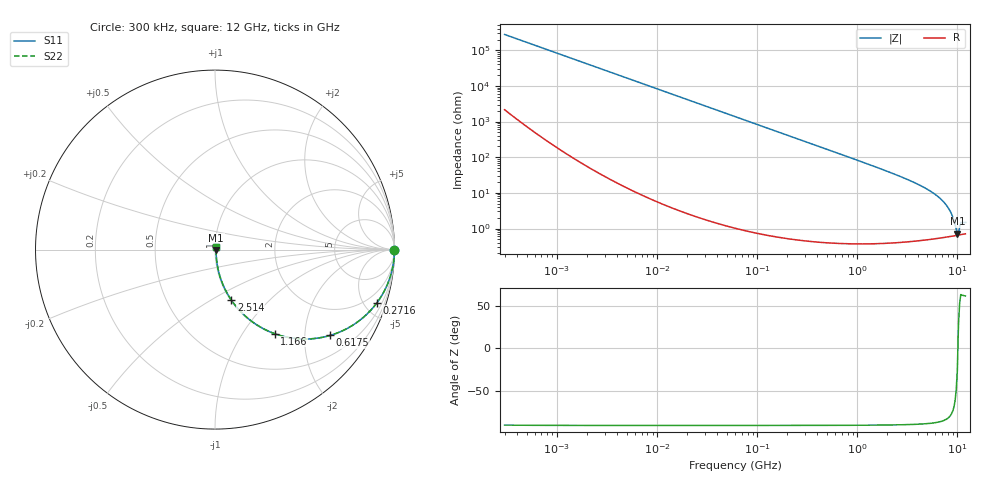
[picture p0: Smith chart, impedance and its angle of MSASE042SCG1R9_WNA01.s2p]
! MSASE042SCG1R9_WNA01  S-PARAMETER MODEL  ( General Type )
! Model Generated by TAIYO YUDEN Corporation (http://www.ty-top.com)
! Version 1.0
! TAIYO YUDEN Control No. 130801
! Copyright(c) 2013 TAIYO YUDEN CO.,LTD. All Rights Reserved.
! Product Description (link to TY-COMPAS)
! https://ds.yuden.co.jp/TYCOMPAS/or/detail?pn=MSASE042SCG1R9AWNA01&u=M
! Products Name : Multilayer Ceramic Capacitors
! Characteristics :
!  Capacitance : 1.9 pF , Rated Voltage : 16V , TCC : CG / C0G
!  Case Size : 0.4 x 0.2 / 0.016 x 0.008 [mm/inch] , Thickness : 0.2 / 0.008 [mm/inch]
!  (Conditions: Temperature = 25 degC , DC Bias Current/Voltage = 0A / 0V)
! External Node Assignments :
!  1  o---| |---o  2
! GND o---------o GND
! Frequency Range : 0.3MHz  -  12000MHz  [ 401 STEP ]
# MHz S RI R 50
! Freq[MHz].  S11 Real  S11 Imag  S21 Real  S21 Imag  S12 Real  S12 Imag  S22 Real  S22 Imag
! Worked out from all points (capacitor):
!   401 points, 300 kHz to 12 GHz, reference 50 ohm
!   read as one part in series: C = 1.92 pF near 316.3 kHz
!   lowest |Z| = 718 mohm at 9.969 GHz (marker M1)
!   series resonance near 10.1 GHz, so ESL is about 130 pH
!   S11 on the Smith chart (normalised r, x): 300 kHz: open; 271.6 MHz: 1.01, -6.11; 617.5 MHz: 1.01, -2.68; 1.166 GHz: 1.01, -1.41; 2.514 GHz: 1.01, -0.62; 12 GHz: 1.01, +0.03
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0.3  1 -0.000361  2.92e-06 0.000361  2.92e-06 0.000361  1 -0.000361
1.769972  1 -0.00213  7.59e-06 0.00213  7.59e-06 0.00213  1 -0.00213
10.44266  0.9998 -0.0126  0.000166 0.0126  0.000166 0.0126  0.9998 -0.0126
60  0.9948 -0.0718  0.00524 0.0718  0.00524 0.0718  0.9948 -0.0718
132.8329  0.9749 -0.1558  0.0251 0.1558  0.0251 0.1558  0.9749 -0.1558
271.6094  0.903 -0.2952  0.097 0.2952  0.097 0.2952  0.903 -0.2952
353.9943  0.8456 -0.3604  0.1544 0.3604  0.1544 0.3604  0.8456 -0.3604
617.4538  0.6422 -0.4779  0.3578 0.4779  0.3578 0.4779  0.6422 -0.4779
848.5281  0.4861 -0.4979  0.5139 0.4979  0.5139 0.4979  0.4861 -0.4979
1166.079  0.3318 -0.4682  0.6682 0.4682  0.6682 0.4682  0.3318 -0.4682
2088.533  0.1293 -0.3305  0.8707 0.3305  0.8707 0.3305  0.1293 -0.3305
2514.07  0.0908 -0.281  0.9092 0.281  0.9092 0.281  0.0908 -0.281
4502.883  0.0258 -0.1437  0.9742 0.1437  0.9742 0.1437  0.0258 -0.1437
6699.894  0.0102 -0.0689  0.9898 0.0689  0.9898 0.0689  0.0102 -0.0689
7448.838  0.0082 -0.0508  0.9918 0.0508  0.9918 0.0508  0.0082 -0.0508
8281.503  0.00697 -0.0331  0.993 0.0331  0.993 0.0331  0.00697 -0.0331
8966.534  0.00649 -0.0201  0.9935 0.0201  0.9935 0.0201  0.00649 -0.0201
9708.23  0.00638 -0.00718  0.9936 0.00718  0.9936 0.00718  0.00638 -0.00718
9968.853  0.00642 -0.00312  0.9936 0.00312  0.9936 0.00312  0.00642 -0.00312
10511.28  0.00665 0.00861  0.9933 -0.00861  0.9933 -0.00861  0.00665 0.00861
11083.22  0.00692 0.0128  0.9931 -0.0128  0.9931 -0.0128  0.00692 0.0128
12000  0.00721 0.0128  0.9928 -0.0128  0.9928 -0.0128  0.00721 0.0128
